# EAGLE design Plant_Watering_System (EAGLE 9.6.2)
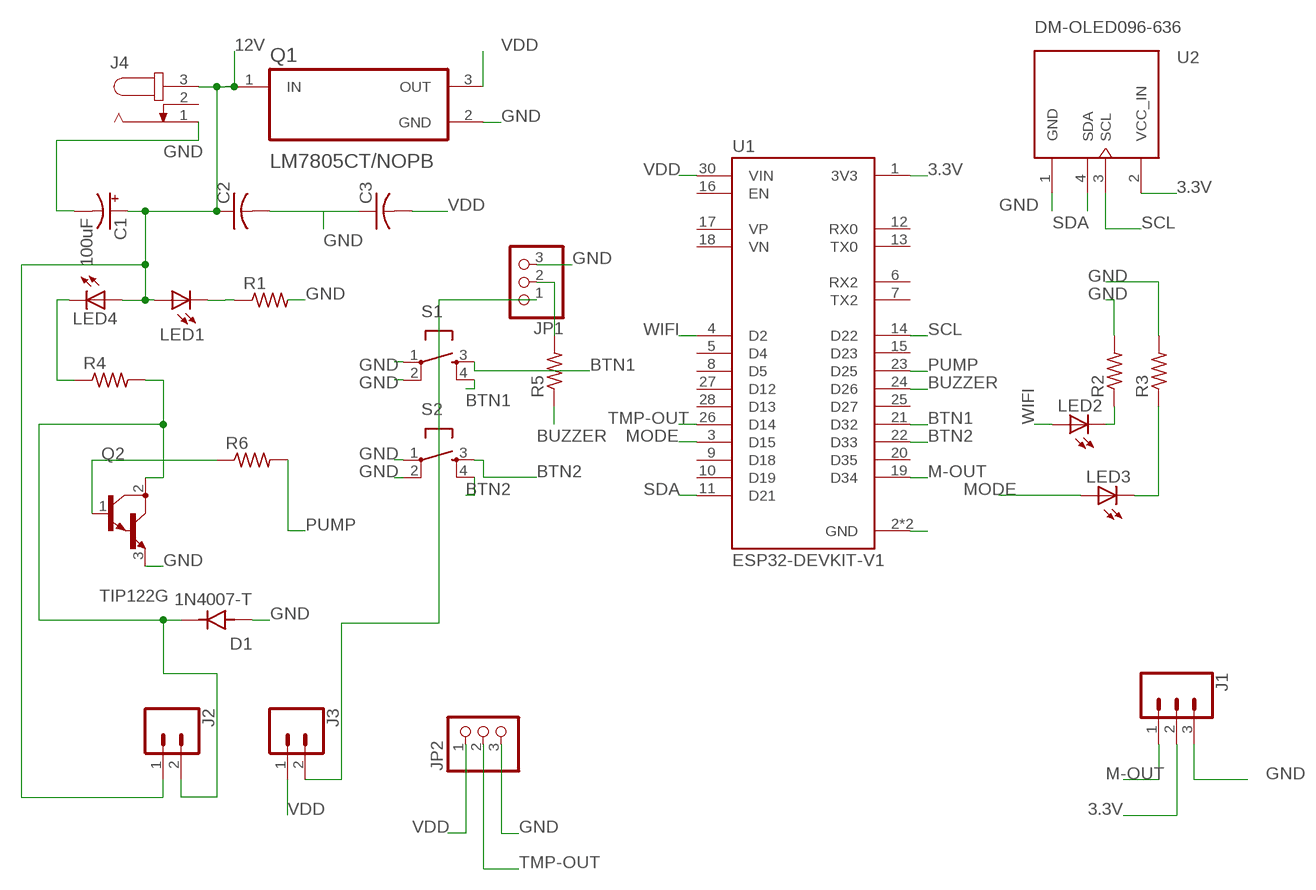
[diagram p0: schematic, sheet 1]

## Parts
C1  100uF  100UF-POLAR-RADIAL-2.5MM-25V-20%  [CPOL-RADIAL-2.5MM-6.5MM]
C2  C-US050-025X075  [C050-025X075]
C3  C-US050-025X075  [C050-025X075]
D1  1N4007-T  [DIOAD780W78L463D236]
J1  CONN_03-SCREW-5MM  [SCREWTERMINAL-5MM-3]
J2  CONN_025MM  [SCREWTERMINAL-5MM-2]
J3  CONN_025MM  [SCREWTERMINAL-5MM-2]
J4  JACK-PLUG1  [SPC4078]
JP1  PINHD-1X3  [1X03]
JP2  PINHD-1X3  [1X03]
LED1  LED5MM  [LED5MM]
LED2  LED5MM  [LED5MM]
LED3  LED5MM  [LED5MM]
LED4  LED5MM  [LED5MM]
Q1  LM7805CT/NOPB  [TO254P1054X470X1955-3]
Q2  TIP122G  [TO254P1009X445X1985-3]
R1  R-US_0309/10  [0309/10]
R2  R-US_0309/10  [0309/10]
R3  R-US_0309/10  [0309/10]
R4  R-US_0309/10  [0309/10]
R5  R-US_0309/10  [0309/10]
R6  R-US_0309/10  [0309/10]
S1  TAC_SWITCHPTH  [TACTILE-PTH]
S2  TAC_SWITCHPTH  [TACTILE-PTH]
U1  ESP32-DEVKIT-V1  [MODULE_ESP32_DEVKIT_V1]
U2  DM-OLED096-636  [MODULE_DM-OLED096-636]

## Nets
3.3V: J1.2 U1.1(3V3) U2.2(VCC_IN)
12V: C1.1(+) C2.1 J2.1 J4.3 LED1.A LED4.A Q1.1(IN)
BTN1: S1.3 S1.4 U1.21(D32)
BTN2: S2.3 S2.4 U1.22(D33)
BUZZER: R5.1 U1.24(D26)
GND: C1.2(-) C2.2 C3.1 D1.A J1.3 J4.1 JP1.3 JP2.3 Q1.2(GND) Q2.3(E) R1.2 R2.2 R3.2 S1.1 S1.2 S2.1 S2.2 U1.2(GND) U1.29(GND) U2.1(GND)
M-OUT: J1.1 U1.19(D34)
MODE: LED3.A U1.3(D15)
N$2: JP1.2 R5.2
N$3: LED1.K(C) R1.1
N$4: LED2.K(C) R2.1
N$5: LED4.K(C) R4.1
N$6: D1.K J2.2 Q2.2(C) R4.2
N$7: Q2.1(B) R6.1
N$11: J3.2 JP1.1
N$14: LED3.K(C) R3.1
PUMP: R6.2 U1.23(D25)
SCL: U1.14(D22) U2.3(SCL)
SDA: U1.11(D21) U2.4(SDA)
TMP-OUT: JP2.2 U1.26(D14)
VDD: C3.2 J3.1 JP2.1 Q1.3(OUT) U1.30(VIN)
WIFI: LED2.A U1.4(D2)
Unconnected: J4.2 U1.5(D4) U1.6(RX2) U1.7(TX2) U1.8(D5) U1.9(D18) U1.10(D19) U1.12(RX0) U1.13(TX0) U1.15(D23) U1.16(EN) U1.17(VP) U1.18(VN) U1.20(D35) U1.25(D27) U1.27(D12) U1.28(D13)

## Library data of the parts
C1 = SparkFun-Capacitors:100UF-POLAR: 100µF polarized capacitors; PROD_ID: CAP-08439
C2 C3 = rcl:C-US: CAPACITOR, American symbol; SPICEPREFIX: C
D1 = 1N4007-T:1N4007-T: Check availability Check availability Check availability; AVAILABILITY: In Stock; CHECK_PRICES: https://www.snapeda.com/parts/1N4007/NTE+Electronics/view-part/?ref=eda; DESCRIPTION: Rectifier Silicon, 1000V, 1 A, DO-41 Case, Solder Leads, 1N Series | NTE Electronics Inc. 1N4007; MF: NTE Electronics, Inc.; MP: 1N4007; PACKAGE: DO-41 NTE Electronics; PRICE: None; SNAPEDA_LINK: https://www.snapeda.com/parts/1N4007/NTE+Electronics/view-part/?ref=snap
J1 = SparkFun-Connectors:CONN_03: Multi connection point. Often used as Generic Header-pin footprint for 0.1 inch spaced/style header connections On any of the 0.1 inch spaced packages, you can populate with these: Break Away Headers - Straight (PRT-00116) Break Away Male Headers - Right Angle (PRT-00553) Female Headers (PRT-00115)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; PROD_ID: CONN-10134; SF_SKU: PRT-08433
J2 J3 = SparkFun-Connectors:CONN_02: Multi connection point. Often used as Generic Header-pin footprint for 0.1 inch spaced/style header connections; SF_SKU: PRT-08432
J4 = con-jack:JACK-PLUG: DC POWER JACK Power Jack, DC, Right Angle, Through Hole, Rated 5A at 16VDC, PC Terminals Distributor: Farnell (www.Farnell.de) Drawing: 84N1161.pdf / 84N1162.pdf Manufacturer: SPC Technology (www.spctechnology.com) Type: SPC4077 / SPC 4078; OC_FARNELL: unknown; OC_NEWARK: unknown
JP1 JP2 = adafruit:PINHD-1X3: PIN HEADER
LED1-LED4 = adafruit:LED: LED
Q1 = LM7805CT_NOPB:LM7805CT/NOPB: Check availability; AVAILABILITY: In Stock; CHECK_PRICES: https://www.snapeda.com/parts/LM7805CT/Texas+Instruments/view-part/?ref=eda; DESCRIPTION: 1.5-A, 35-V, linear voltage regulator 3-TO-220 0 to 125; MF: Texas Instruments; MP: LM7805CT; PACKAGE: TO-220-3 Texas Instruments; PRICE: None; SNAPEDA_LINK: https://www.snapeda.com/parts/LM7805CT/Texas+Instruments/view-part/?ref=snap
Q2 = TIP122G:TIP122G: Bipolar (BJT) Transistor NPN - Darlington 100V 5A 2W Through Hole TO-220AB Check availability; AVAILABILITY: Not in stock; CHECK_PRICES: https://www.snapeda.com/parts/TIP122G/Rochester+Electronics/view-part/?ref=eda; DESCRIPTION: Bipolar (BJT) Transistor NPN - Darlington 100V 5A 2W Through Hole TO-220AB; MF: Rochester Electronics, LLC; MP: TIP122G; PACKAGE: Package; PRICE: None; SNAPEDA_LINK: https://www.snapeda.com/parts/TIP122G/Rochester+Electronics/view-part/?ref=snap
R1-R6 = rcl:R-US_: RESISTOR, American symbol; SPICEPREFIX: R
S1 S2 = SparkFun-Retired:TAC_SWITCH: Momentary Switch Button commonly used for reset or general input. Spark Fun Electronics SKU : COM-00097 SMT- SWCH-08247
U1 = ESP32-DEVKIT-V1:ESP32-DEVKIT-V1: Dual core, Wi-Fi: 2.4 GHz up to 150 Mbits/s,BLE (Bluetooth Low Energy) and legacy Bluetooth, 32 bits, Up to 240 MHz Check availability; AVAILABILITY: Not in stock; CHECK_PRICES: https://www.snapeda.com/parts/ESP32-DEVKIT-V1/Do+it/view-part/?ref=eda; DESCRIPTION: Dual core, Wi-Fi: 2.4 GHz up to 150 Mbits/s,BLE (Bluetooth Low Energy) and legacy Bluetooth, 32 bits, Up to 240 MHz; MF: Do it; MP: ESP32-DEVKIT-V1; PACKAGE: None; PRICE: None; SNAPEDA_LINK: https://www.snapeda.com/parts/ESP32-DEVKIT-V1/Do+it/view-part/?ref=snap
U2 = DM-OLED096-636:DM-OLED096-636: Check availability; AVAILABILITY: Not in stock; CHECK_PRICES: https://www.snapeda.com/parts/DM-OLED096-636/Display+Module/view-part/?ref=eda; DESCRIPTION: 0.96” 128 X 64 MONOCHROME GRAPHIC OLED DISPLAY MODULE - I2C; MF: Display Module; MP: DM-OLED096-636; PACKAGE: Package; PRICE: None; SNAPEDA_LINK: https://www.snapeda.com/parts/DM-OLED096-636/Display+Module/view-part/?ref=snap

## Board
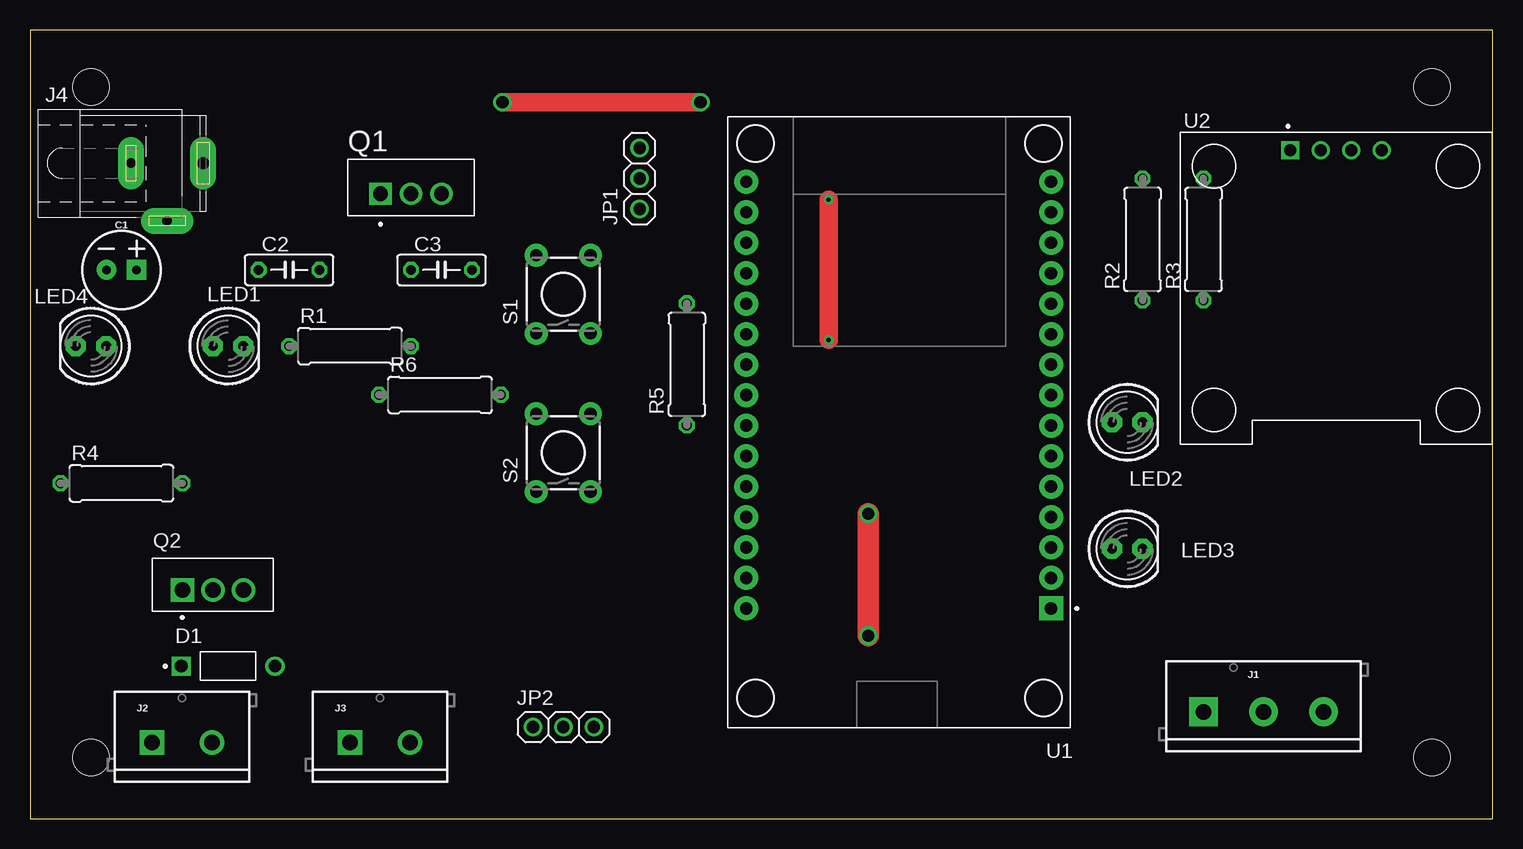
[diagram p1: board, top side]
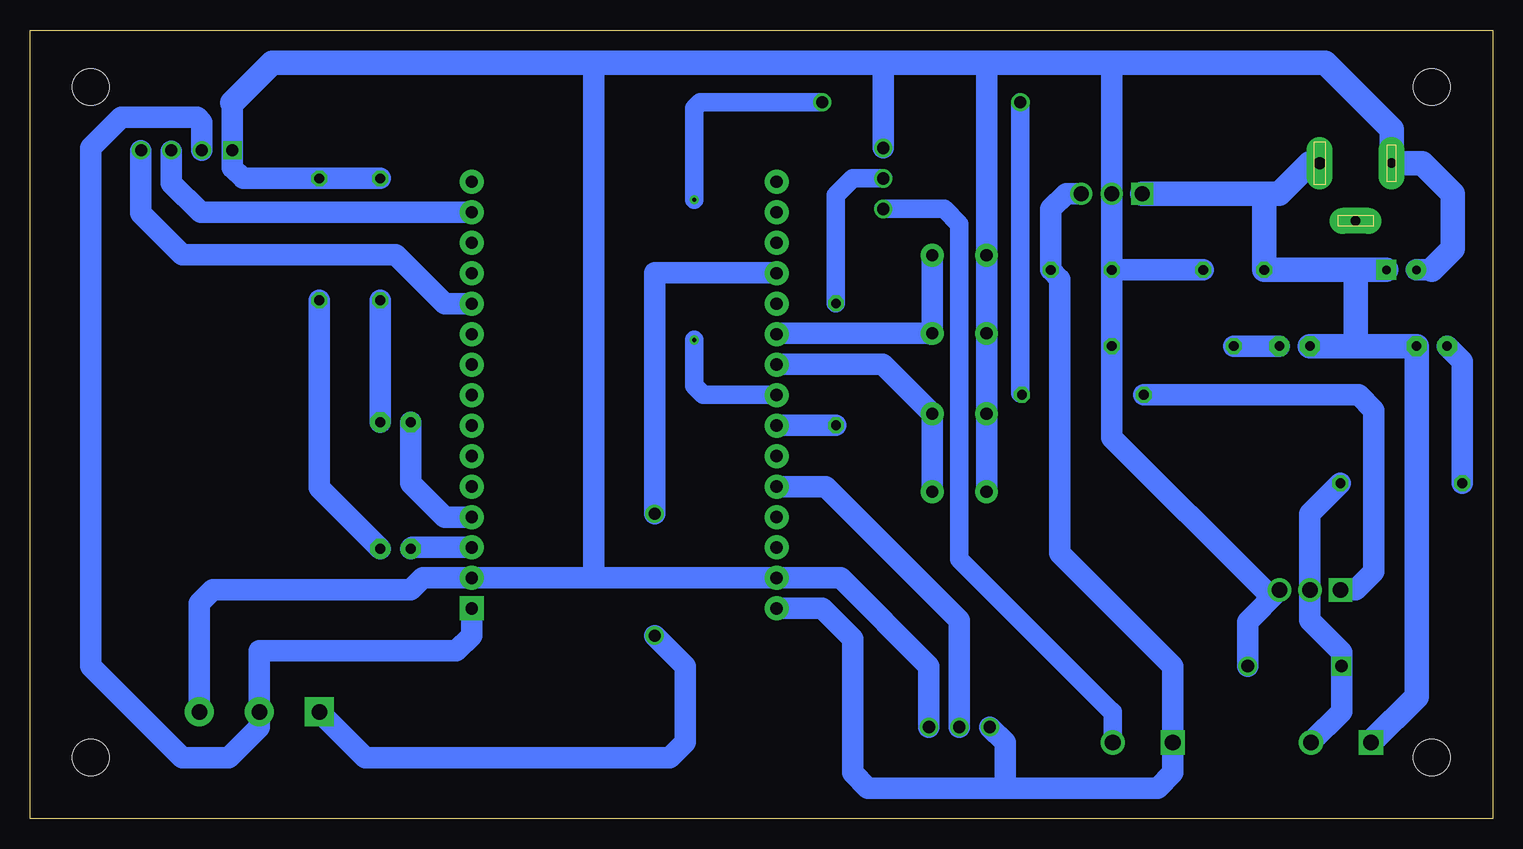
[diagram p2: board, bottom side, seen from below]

Size 121.9 x 65.71 mm. Coordinates in mm from the lower left corner, seen from the top.
Outline: 0,0 121.9,0 121.9,65.71 0,65.71 0,0
Copper layers (1*16): Top 0.035mm / dielectric 1.5mm / Bottom 0.035mm
Design rules "default": minimum track width 6mil, minimum drill 0.35mm, track to track 6mil, track to pad 6mil, pad to pad 6mil, via to via 6mil, smd to smd 6mil, copper to edge 40mil, drill to drill 6mil, minimum pad ring 10mil, minimum via ring 8mil, stop-mask expansion 4mil, vias tented up to drill 0mil, thermal gap 10mil
Holes 3.05 mm at 5.08,60.96 116.84,60.96 116.84,5.08 5.08,5.08

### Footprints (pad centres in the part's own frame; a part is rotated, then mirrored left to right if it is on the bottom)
CPOL-RADIAL-2.5MM-6.5MM = drill 0.7 pad 1.651 square: 1 1.25,0 | drill 0.7 pad 1.651: 2 -1.25,0
C050-025X075 = drill 0.813 octagon: 1 -2.54,0; 2 2.54,0
DIOAD780W78L463D236 = drill 1.06: A 3.905,0 | drill 1.06 square: K -3.905,0
SCREWTERMINAL-5MM-3 = drill 1.3 pad 2.413 square: 1 0,0 | drill 1.3 pad 2.413: 2 5,0; 3 10,0
SCREWTERMINAL-5MM-2 = drill 1.3 pad 2.032 square: 1 0,0 | drill 1.3 pad 2.032: 2 5,0
SPC4078 = drill 0.8 pad 2.184 long: 1 -3,0; 2 0,-4.8 | drill 1 pad 2.184 long: 3 3,0
1X03 = drill 1.016: 1 -2.54,0; 2 0,0; 3 2.54,0
LED5MM = drill 0.813 pad 1.676 octagon: A -1.27,0; K 1.27,0
TO254P1054X470X1955-3 = drill 1.24 square: 1 -2.54,0 | drill 1.24: 2 0,0; 3 2.54,0
TO254P1009X445X1985-3 = drill 1.29 pad 1.94 square: 1 -2.54,0 | drill 1.29 pad 1.94: 2 0,0; 3 2.54,0
0309/10 = drill 0.813 octagon: 1 -5.08,0; 2 5.08,0
TACTILE-PTH = drill 1.016 pad 1.88: 1 -3.251,2.261; 2 3.251,2.261; 3 -3.251,-2.261; 4 3.251,-2.261
MODULE_ESP32_DEVKIT_V1 = drill 1.02 pad 2 square: 1 -12.7,15.515 | drill 1.02 pad 2: 2 -12.7,12.975; 3 -12.7,10.435; 4 -12.7,7.895; 5 -12.7,5.355; 6 -12.7,2.815; 7 -12.7,0.275; 8 -12.7,-2.265; 9 -12.7,-4.805; 10 -12.7,-7.345; 11 -12.7,-9.885; 12 -12.7,-12.425; 13 -12.7,-14.965; 14 -12.7,-17.505; 15 -12.7,-20.045; 16 12.7,-20.045; 17 12.7,-17.505; 18 12.7,-14.965; 19 12.7,-12.425; 20 12.7,-9.885; 21 12.7,-7.345; 22 12.7,-4.805; 23 12.7,-2.265; 24 12.7,0.275; 25 12.7,2.815; 26 12.7,5.355; 27 12.7,7.895; 28 12.7,10.435; 29 12.7,12.975; 30 12.7,15.515
MODULE_DM-OLED096-636 = drill 1 square: 1 -3.81,11.5 | drill 1: 2 -1.27,11.5; 3 1.27,11.5; 4 3.81,11.5

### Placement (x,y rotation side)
C1  7.62,45.72 0 top
C2  21.59,45.72 0 top
C3  34.29,45.72 0 top
D1  16.51,12.7 0 top
J1  97.79,8.89 0 top
J2  10.16,6.35 0 top
J3  26.67,6.35 0 top
J4  11.43,54.61 0 top
JP1  50.8,53.34 90 top
JP2  44.45,7.62 0 top
LED1  16.51,39.37 0 top
LED2  91.44,33.02 0 top
LED3  91.44,22.48 0 top
LED4  5.08,39.37 180 top
Q1  31.75,52.07 0 top
Q2  15.24,19.05 0 top
R1  26.67,39.37 0 top
R2  92.71,48.26 90 top
R3  97.79,48.26 90 top
R4  7.62,27.94 0 top
R5  54.74,37.85 90 top
R6  34.16,35.31 0 top
S1  44.45,43.69 90 top
S2  44.45,30.48 90 top
U1  72.39,33.02 180 top
U2  108.84,44.2 0 top

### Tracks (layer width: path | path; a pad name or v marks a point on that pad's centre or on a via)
3.3V
  Bottom 0.152: U2.2 107.57,58.04
  Bottom 1.778: 107.57,55.68 107.57,58.04 107.95,58.42 114.3,58.42 116.84,55.88 116.84,12.7 109.22,5.08 105.33,5.08 102.79,7.62 J1.2 102.79,13.97 86.36,13.97 85.09,15.24 U1.1
12V
  Bottom 1.778: 11.43,39.37 LED1.A
  Bottom 2.032: Q1.1 19.05,52.07 | 19.05,52.07 17.78,52.07 15.24,54.61 J4.3 | 19.05,52.07 C2.1 | 19.05,46.99 C2.1 | C1.1 11.43,45.72 | 11.43,45.72 | 11.43,39.37 11.43,45.72 | LED1.A LED4.A 6.35,10.16 J2.1 | C2.1 11.43,45.72
BTN1
  Bottom 0.152: U1.21 59.62,40.44
  Bottom 1.778: S1.3 46.78,40.37 | S1.4 S1.3 | 59.62,40.44 S1.3
BTN2
  Bottom 0.152: U1.22 59.67,37.85
  Bottom 1.778: 59.67,37.85 50.83,37.85 S2.4 S2.3
BUZZER
  Bottom 0.152: U1.24 59.67,32.77
  Bottom 1.778: 59.67,32.77 R5.1
GND
  Bottom 0.152: 74.17,62.99 74.93,62.23 74.93,62.99 | 42.19,62.71 41.91,62.99 | 19.05,19.05 Q2.3 | U1.2 85.11,20.07 | 105.05,59.67 105.06,59.66 | 105.06,54.26 105.03,54.23 U2.1
  Bottom 1.778: S2.1 S2.2 S1.1 S1.2 42.19,62.71 | JP2.3 46.99,12.7 54.34,20.05 U1.29 74.93,20.05 | 5.1,45.72 C1.2 | R2.2 R3.2 104.14,53.34 105.03,54.23 | JP1.3 50.8,62.99 | 31.75,62.99 Q1.2 C3.1 | C3.1 R1.2 31.75,31.75 19.05,19.05 | Q2.3 20.41,16.42 D1.A | J1.3 107.79,17.94 106.68,19.05 90.17,19.05 89.15,20.07 85.11,20.07 | 74.93,20.05 U1.2 | 74.93,20.05 74.93,62.23 | C2.2 C3.1 | 105.06,59.66 105.06,54.26
  Bottom 2.032: 105.05,59.67 101.73,62.99 74.93,62.99 50.8,62.99 41.91,62.99 31.75,62.99 13.97,62.99 8.43,57.45 J4.1 5.89,54.61 3.35,52.07 3.35,47.47 5.1,45.72
M-OUT  (via drill 1.02)
  Top 1.778: v69.85,15.24 v69.85,25.4
  Bottom 0.152: 59.71,45.47 U1.19
  Bottom 1.778: J1.1 93.98,5.08 68.58,5.08 67.31,6.35 67.31,12.7 v69.85,15.24 | v69.85,25.4 69.85,45.47 59.71,45.47
MODE
  Bottom 0.152: LED3.A 90.04,22.61 | U1.3 85.11,22.61
  Bottom 1.778: LED3.A 90.06,22.59 | 90.04,22.61 85.11,22.61
N$2
  Bottom 1.524: JP1.2 53.34,53.34 54.74,51.94 R5.2
N$3
  Bottom 1.778: LED1.K R1.1
N$4
  Bottom 1.778: R2.1 LED2.K
N$5
  Bottom 1.778: LED4.K 2.54,38.1 R4.1
N$6
  Bottom 0.152: 15.24,16.61 12.61,13.97 D1.K | Q2.2 15.24,16.51
  Bottom 1.778: 15.24,16.61 15.24,25.4 R4.2 | J2.2 12.61,8.9 D1.K 12.61,13.88 15.24,16.51
N$7
  Bottom 1.778: Q2.1 11.43,19.05 9.91,20.57 9.91,34.04 11.18,35.31 R6.1
N$11
  Bottom 1.524: J3.2 31.67,8.89 31.71,8.85 44.45,21.59 44.45,49.53 45.72,50.8 JP1.1
N$14
  Bottom 1.778: R3.1 97.79,27.56 LED3.K
PUMP  (via drill 0.35, 1.02)
  Top 1.524: v39.37,59.69 v55.88,59.69 | v66.55,39.88 v66.55,51.56
  Bottom 0.152: 39.37,35.43 R6.2 | U1.23 59.71,35.31
  Bottom 1.524: v55.88,59.69 66.04,59.69 66.55,59.18 v66.55,51.56 | 59.71,35.31 65.79,35.31 66.55,36.07 v66.55,39.88 | v39.37,59.69 39.37,35.43
SCL
  Bottom 0.152: U2.3 110.11,52.96
  Bottom 1.778: 110.11,55.62 110.11,52.96 107.67,50.52 U1.14
SDA
  Bottom 0.152: 112.65,50.48 112.68,50.45 | 112.68,55.66 U2.4
  Bottom 1.778: U1.11 87.36,42.91 91.44,46.99 109.22,46.99 112.68,50.45 112.68,55.66
TMP-OUT
  Bottom 1.778: JP2.2 44.45,16.51 55.6,27.66 U1.26
VDD
  Bottom 1.778: 40.64,2.54 27.94,2.54 26.67,3.81 J3.1 26.67,12.7 36.07,22.1 36.07,44.96 C3.2 36.83,50.8 35.56,52.07 Q1.3 | 40.64,2.54 52.07,2.54 53.34,3.81 53.34,14.96 55.88,17.5 U1.30 | JP2.1 40.64,6.35 40.64,2.54
WIFI
  Bottom 1.778: LED2.A 90.17,27.94 87.36,25.12 U1.4

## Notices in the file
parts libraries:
SparkFun-Capacitors: Licensing: Creative Commons ShareAlike 4.0 International - https://creativecommons.org/licenses/by-sa/4.0
